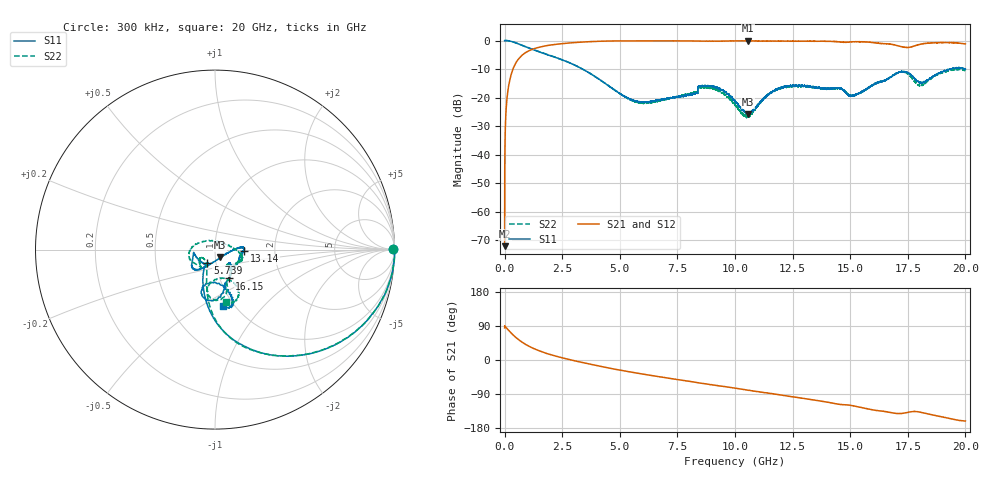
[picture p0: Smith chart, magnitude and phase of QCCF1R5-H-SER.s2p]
!QCCF1R5
!Johanson Technology Inc.
!www.johansontechnology.com
!Test Board Conditions:
!Substrate Type  RO4350B
!Substrate Thickness  10 mil
!Substrate Dk  3.66
!TL Type: GCPW
!TL Trace Width  21 mil
!TL Gap  20 mil
!Electrode orientation  Horizontal
!DUT TOPOLOGY	SERIES
!Mounting Pad LxW  16x21 mil
# MHz S  dB  R 50
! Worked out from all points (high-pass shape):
!   20001 points, 300 kHz to 20 GHz, reference 50 ohm
!   highest |S21| = -0.09 dB at 10.55 GHz (marker M1); lowest = -72.0 dB at 300 kHz (marker M2)
!   |S21| within 3 dB of the highest: 1.204032 GHz to 1.204782 GHz (750 kHz wide, 0.0623 % of centre); 1.206 GHz to end of sweep
!   lowest |S11| = -25.8 dB at 10.57 GHz (marker M3), VSWR 1.11, Z = 52.8 - j4.5 ohm
!   |S11| at or under -10 dB: 3.382 GHz to 19.31 GHz (15.93 GHz wide, 140 % of centre); 19.31081 GHz to 19.31244 GHz (1.632 MHz wide, 0.00845 % of centre); 19.98778 GHz to end of sweep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
!   |S22| runs from -27.0 to 0.0 dB; largest |S21 - S12| = 0.026
!   S11 on the Smith chart (normalised r, x): 300 kHz: open; 5.739 GHz: 0.91, -0.14; 13.14 GHz: 1.38, -0.03; 16.15 GHz: 1.11, -0.37; 20 GHz: 0.89, -0.61
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0.3  -0.06 0.2  -72.05 84.9  -70.58 66.8  -0.06 0.2
101.298  -0.03 -6.6  -20.50 83.2  -20.52 83.3  -0.03 -6.6
128.298  -0.06 -8.4  -18.49 81.3  -18.50 81.4  -0.06 -8.5
256.296  -0.25 -16.4  -12.72 73.0  -12.72 73.3  -0.26 -16.5
470.293  -0.77 -28.8  -8.10 60.5  -8.09 60.7  -0.79 -28.8
1559.277  -4.14 -66.8  -2.25 23.1  -2.24 22.8  -4.06 -66.4
3334.25  -9.79 -96.7  -0.56 -6.1  -0.57 -6.0  -9.81 -94.8
5739.214  -21.31 -119.8  -0.13 -34.6  -0.13 -34.6  -21.67 -128.4
6667.2  -20.92 -117.4  -0.14 -43.8  -0.13 -43.7  -21.23 -149.6
8654.17  -15.91 -141.9  -0.21 -62.4  -0.21 -62.3  -16.52 -162.6
10000.15  -21.09 -109.4  -0.13 -74.4  -0.15 -74.2  -22.57 143.1
10548.14  -25.27 -59.2  -0.09 -79.4  -0.13 -79.2  -26.30 73.2
10574.14  -25.80 -55.9  -0.12 -79.9  -0.12 -79.5  -26.38 69.2
11720.12  -17.61 4.2  -0.21 -89.7  -0.21 -90.2  -17.68 -5.6
13135.1  -15.83 -3.1  -0.25 -102.8  -0.21 -102.5  -15.99 -24.5
13334.1  -16.30 -5.7  -0.26 -104.7  -0.28 -104.8  -16.35 -24.4
15060.07  -19.48 -43.3  -0.49 -120.3  -0.45 -119.8  -19.52 -49.6
16146.06  -14.97 -64.0  -0.90 -133.3  -0.86 -133.0  -14.77 -65.3
16667.05  -13.40 -76.1  -1.21 -137.6  -1.20 -138.2  -13.19 -71.8
17328.04  -10.87 -97.1  -2.33 -140.5  -2.44 -140.0  -11.11 -91.4
18081.03  -14.64 -92.9  -1.24 -138.4  -1.26 -137.5  -15.65 -77.9
20000  -10.07 -82.3  -1.19 -160.9  -1.04 -159.9  -10.51 -78.3
